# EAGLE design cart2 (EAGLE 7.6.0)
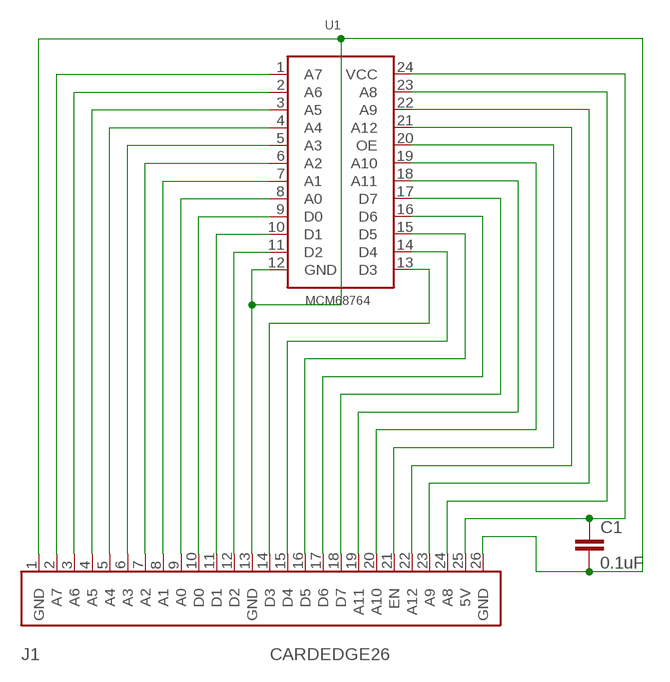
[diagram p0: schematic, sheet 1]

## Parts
C1  0.1uF  C-EU150-054X183  [C150-054X183]
J1  CARDEDGE26  [CARDEDGE26]
U1  MCM68764  [DIL24]

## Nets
GND: C1.2 J1.1(GND) J1.13(GND) J1.26(GND) U1.12(GND)
N$2: J1.2(A7) U1.1(A7)
N$3: J1.3(A6) U1.2(A6)
N$4: J1.4(A5) U1.3(A5)
N$5: J1.5(A4) U1.4(A4)
N$6: J1.6(A3) U1.5(A3)
N$7: J1.7(A2) U1.6(A2)
N$8: J1.8(A1) U1.7(A1)
N$9: J1.9(A0) U1.8(A0)
N$10: J1.10(D0) U1.9(D0)
N$11: J1.11(D1) U1.10(D1)
N$12: J1.12(D2) U1.11(D2)
N$13: J1.14(D3) U1.13(D3)
N$14: J1.15(D4) U1.14(D4)
N$15: J1.16(D5) U1.15(D5)
N$16: J1.17(D6) U1.16(D6)
N$17: J1.18(D7) U1.17(D7)
N$18: J1.19(A11) U1.18(A11)
N$19: J1.20(A10) U1.19(A10)
N$20: J1.21(EN) U1.20(OE)
N$21: J1.22(A12) U1.21(A12)
N$22: J1.23(A9) U1.22(A9)
N$23: J1.24(A8) U1.23(A8)
N$24: C1.1 J1.25(5V) U1.24(VCC)

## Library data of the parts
C1 = rcl:C-EU: CAPACITOR, European symbol
J1 = bally:CARDEDGE26: Bally Astrocade cartridge 26 pin card edge connector.
U1 = bally:MCM68764: Motorola MCM68764 EPROM (8K x 8)

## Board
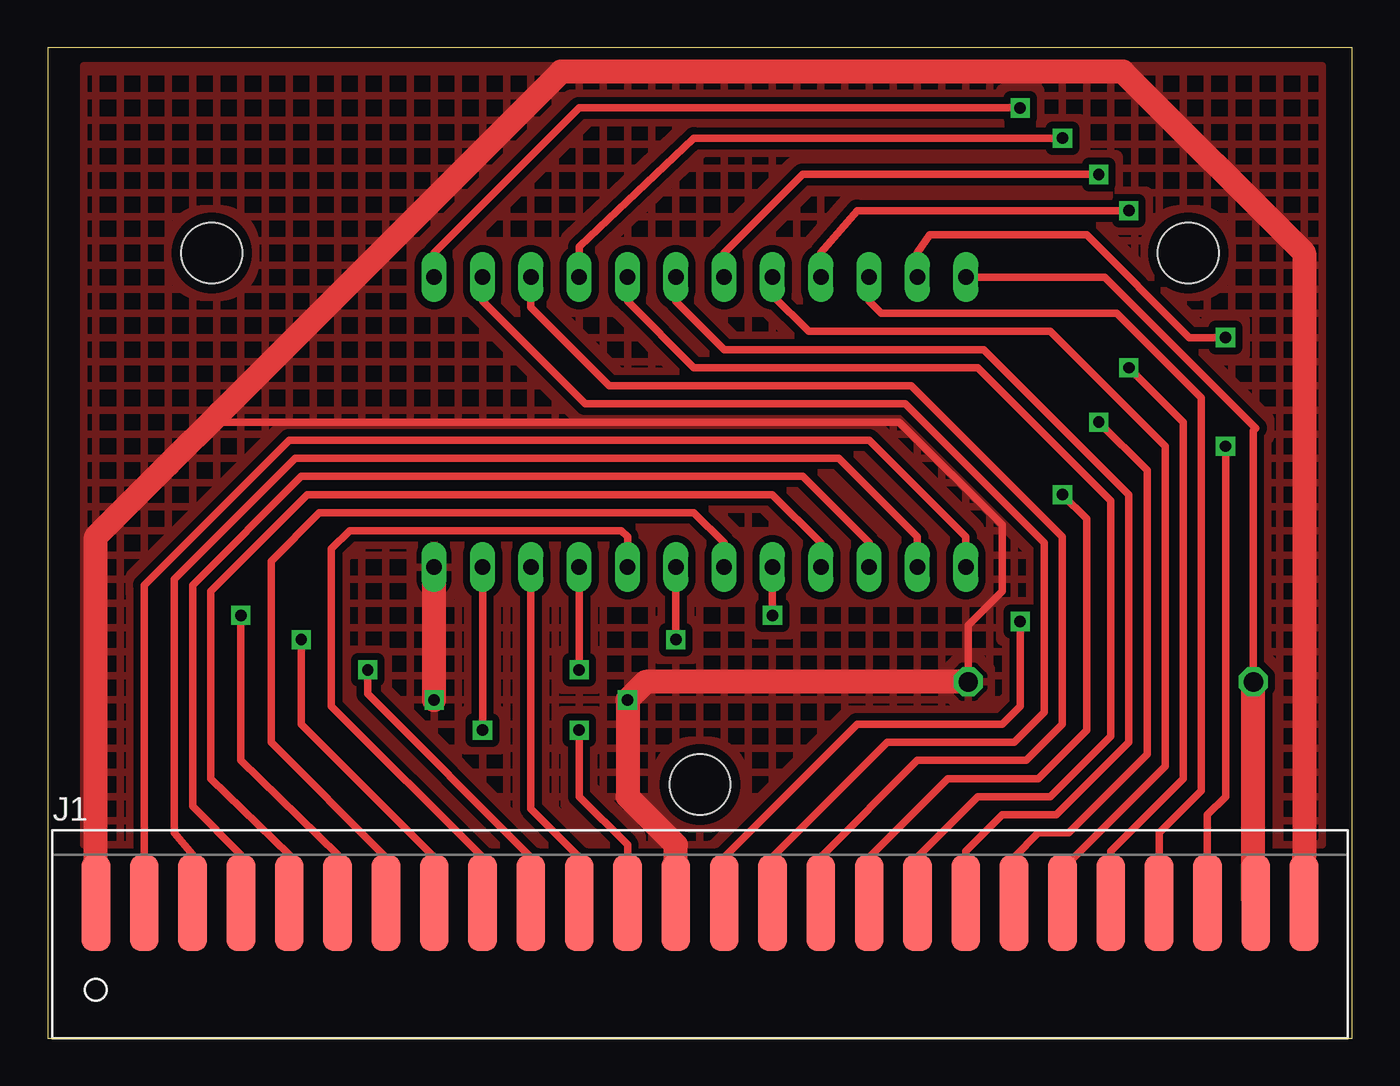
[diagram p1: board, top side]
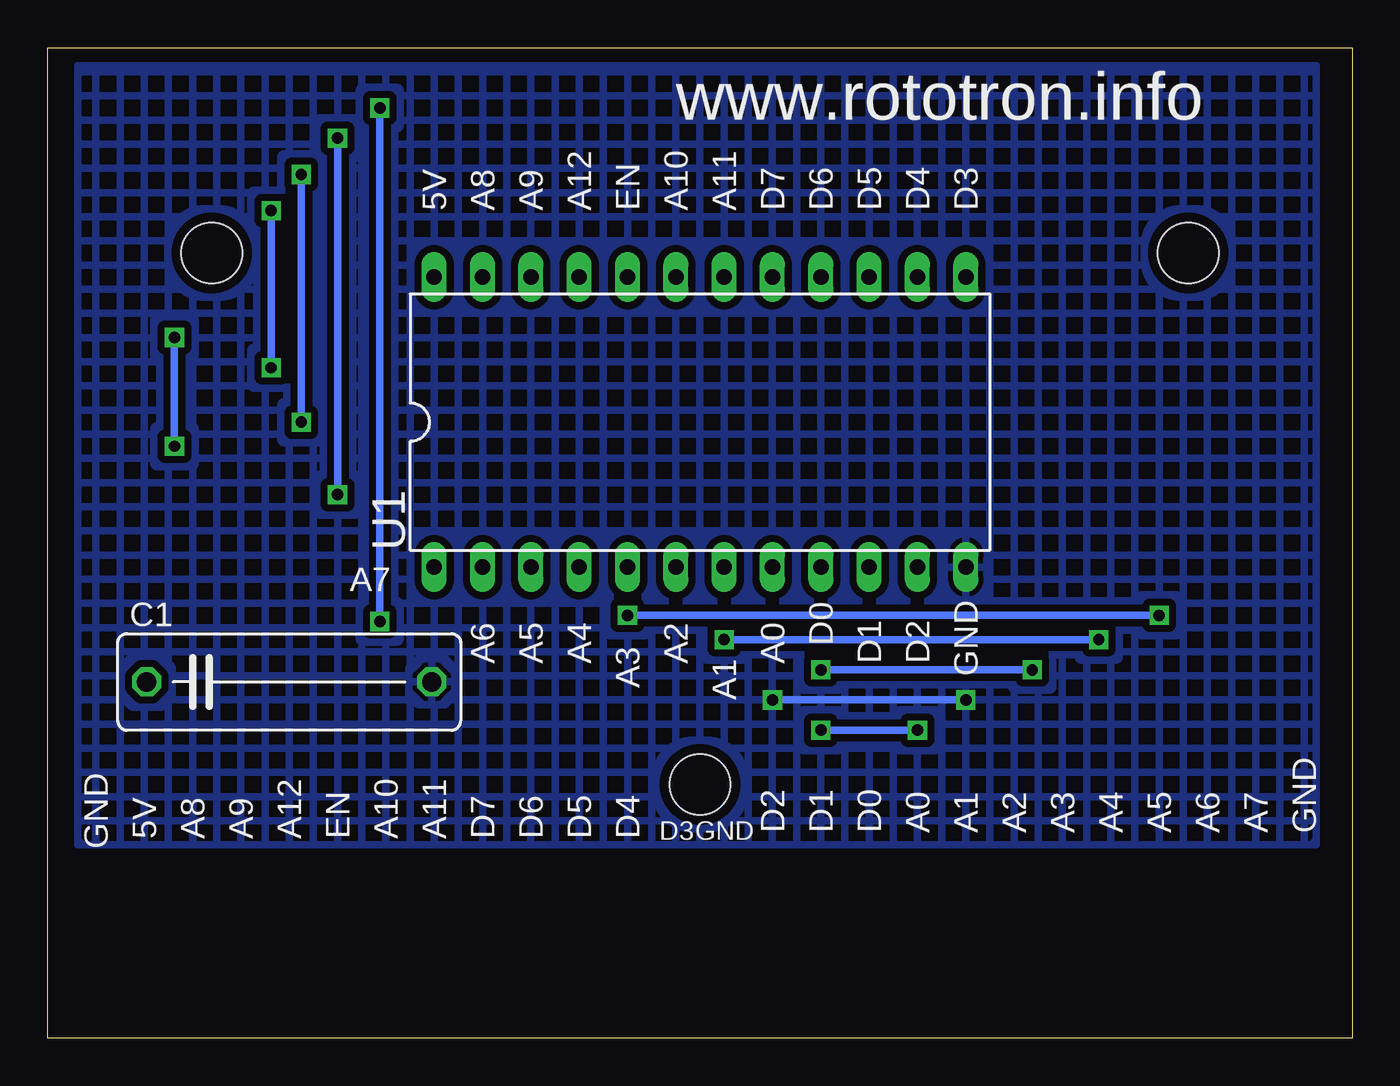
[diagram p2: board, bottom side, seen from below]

Size 68.58 x 52.06 mm. Coordinates in mm from the lower left corner, seen from the top.
Outline: 0,0 68.58,0 68.58,52.06 0,52.06 0,0
Copper layers (1*16): Top 0.035mm / dielectric 1.5mm / Bottom 0.035mm
Design rules "default *": minimum track width 10mil, minimum drill 24mil, track to track 15mil, track to pad 15mil, pad to pad 20mil, via to via 20mil, smd to smd 20mil, copper to edge 20mil, drill to drill 8mil, minimum pad ring 10mil, minimum via ring 8mil, stop-mask expansion 4mil, vias tented up to drill 0mil, thermal gap 10mil
Holes 3.2 mm at 34.29,13.34 8.64,41.27 59.94,41.27

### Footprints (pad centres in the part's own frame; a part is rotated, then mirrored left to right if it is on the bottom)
C150-054X183 = drill 1.016 octagon: 1 -7.493,0; 2 7.493,0
CARDEDGE26 = smd 1.524 x 5.08: 1 2.286,7.112; 2 4.826,7.112; 3 7.366,7.112; 4 9.906,7.112; 5 12.446,7.112; 6 14.986,7.112; 7 17.526,7.112; 8 20.066,7.112; 9 22.606,7.112; 10 25.146,7.112; 11 27.686,7.112; 12 30.226,7.112; 13 32.766,7.112; 14 35.306,7.112; 15 37.846,7.112; 16 40.386,7.112; 17 42.926,7.112; 18 45.466,7.112; 19 48.006,7.112; 20 50.546,7.112; 21 53.086,7.112; 22 55.626,7.112; 23 58.166,7.112; 24 60.706,7.112; 25 63.246,7.112; 26 65.786,7.112
DIL24 = drill 0.813 long: 1 1.27,-0.635; 2 3.81,-0.635; 3 6.35,-0.635; 4 8.89,-0.635; 5 11.43,-0.635; 6 13.97,-0.635; 7 16.51,-0.635; 8 19.05,-0.635; 9 21.59,-0.635; 10 24.13,-0.635; 11 26.67,-0.635; 12 29.21,-0.635; 13 29.21,14.605; 14 26.67,14.605; 15 24.13,14.605; 16 21.59,14.605; 17 19.05,14.605; 18 16.51,14.605; 19 13.97,14.605; 20 11.43,14.605; 21 8.89,14.605; 22 6.35,14.605; 23 3.81,14.605; 24 1.27,14.605

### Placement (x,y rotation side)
C1  55.88,18.73 0 bottom
J1  0.25,0 0 top
U1  49.53,25.4 0 bottom

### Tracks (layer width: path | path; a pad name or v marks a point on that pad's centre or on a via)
GND  (via drill 0.6)
  Top 0.406: 33.02,6.99 J1.13 | 66.04,9.53 J1.26 | 8.57,32.38 44.77,32.38 50.16,26.99 50.16,23.5 48.39,21.72 C1.2 | 8.57,32.38 8.61,32.35 | 8.57,32.38 8.26,32.07 9.05,32.86
  Top 1.27: J1.1 2.54,26.35 6.35,30.16 9.05,32.86 26.99,50.8 56.52,50.8 66.04,41.27 66.04,9.53 | v20.32,17.78 U1.12 | J1.13 33.02,10.16 30.48,12.7 v30.48,17.78 31.43,18.73 C1.2
  Bottom 0.406: v30.48,17.78 v20.32,17.78
  pour Top (hatched): 1.91,10.16 1.91,51.12 66.99,51.12 66.99,10.16
  pour Bottom (hatched): 1.91,10.16 1.91,51.12 66.99,51.12 66.99,10.16
N$2
  Top 0.406: U1.1 48.26,26.35 43.18,31.43 12.7,31.43 5.08,23.81 J1.2
N$3
  Top 0.406: U1.2 45.72,26.35 41.59,30.48 13.02,30.48 6.67,24.13 6.67,10.79 7.62,9.65 J1.3
N$4
  Top 0.406: U1.3 43.18,26.04 39.69,29.53 13.34,29.53 7.62,23.81 7.62,12.19 10.16,9.65 J1.4
N$5
  Top 0.406: U1.4 40.64,26.04 38.1,28.57 13.65,28.57 8.57,23.5 8.57,13.65 12.7,9.65 J1.5
N$6  (via drill 0.6)
  Top 0.406: U1.5 v38.1,22.23 | v10.16,22.23 10.16,14.61 15.24,9.65 J1.6
  Bottom 0.406: v38.1,22.23 v10.16,22.23
N$7
  Top 0.406: U1.6 35.56,26.04 33.97,27.62 14.29,27.62 11.75,25.08 11.75,15.56 17.78,9.53 J1.7
N$8  (via drill 0.6)
  Top 0.406: U1.7 v33.02,20.95 | v13.34,20.95 13.34,16.51 20.32,9.53 J1.8
  Bottom 0.406: v33.02,20.95 v13.34,20.95
N$9
  Top 0.406: U1.8 30.48,26.35 30.16,26.67 15.88,26.67 14.92,25.72 14.92,17.46 22.86,9.53 J1.9
N$10  (via drill 0.6)
  Top 0.406: U1.9 v27.94,19.37 | v16.83,19.37 16.83,18.1 25.4,9.53 J1.10
  Bottom 0.406: v27.94,19.37 v16.83,19.37
N$11
  Top 0.406: U1.10 25.4,12.06 27.94,9.53 J1.11
N$12  (via drill 0.6)
  Top 0.406: J1.12 30.48,10.16 27.94,12.7 v27.94,16.19 | v22.86,16.19 U1.11
  Bottom 0.406: v27.94,16.19 v22.86,16.19
N$13  (via drill 0.6)
  Top 0.406: U1.13 20.32,41.27 27.94,48.9 v51.12,48.9 | v51.12,21.91 51.12,17.46 50.16,16.51 42.55,16.51 35.56,9.53 J1.14
  Bottom 0.406: v51.12,48.9 v51.12,21.91
N$14
  Top 0.406: U1.14 22.86,38.73 28.26,33.34 45.09,33.34 52.39,26.04 52.39,17.14 50.8,15.56 44.13,15.56 38.1,9.53 J1.15
N$15
  Top 0.406: U1.15 25.4,38.42 29.53,34.29 45.4,34.29 53.34,26.35 53.34,16.51 51.44,14.61 45.72,14.61 40.64,9.53 J1.16
N$16  (via drill 0.6)
  Top 0.406: U1.16 27.94,41.59 33.97,47.31 v53.34,47.31 | v53.34,28.57 54.61,27.3 54.61,16.19 52.07,13.65 47.31,13.65 43.18,9.53 J1.17
  Bottom 0.406: v53.34,47.31 v53.34,28.57
N$17
  Top 0.406: U1.17 30.48,38.73 33.97,35.24 48.9,35.24 55.88,28.26 55.88,15.88 52.7,12.7 48.9,12.7 45.72,9.53 J1.18
N$18
  Top 0.406: U1.18 33.02,38.73 35.56,36.2 49.21,36.2 56.83,28.57 56.83,15.56 53.02,11.75 50.16,11.75 48.26,9.84 J1.19
N$19  (via drill 0.6)
  Top 0.406: U1.19 35.56,41.27 39.69,45.4 v55.24,45.4 | v55.24,32.38 57.78,29.84 57.78,14.92 53.66,10.79 52.07,10.79 50.8,9.53 J1.20
  Bottom 0.406: v55.24,45.4 v55.24,32.38
N$20
  Top 0.406: U1.20 38.1,39.05 40.01,37.15 52.7,37.15 58.74,31.11 58.74,14.29 53.34,8.89 J1.21
N$21  (via drill 0.6)
  Top 0.406: U1.21 40.64,41.27 42.55,43.5 v56.83,43.5 | v56.83,35.24 59.69,32.38 59.69,13.65 55.88,9.84 J1.22
  Bottom 0.406: v56.83,43.5 v56.83,35.24
N$22
  Top 0.406: U1.22 43.18,38.73 43.81,38.1 56.2,38.1 60.64,33.66 60.64,13.02 58.42,10.79 J1.23
N$23  (via drill 0.6)
  Top 0.406: U1.23 45.72,41.27 46.35,42.23 54.61,42.23 60.01,36.83 v61.91,36.83 | J1.24 60.96,11.75 61.91,12.7 v61.91,31.11
  Bottom 0.406: v61.91,36.83 v61.91,31.11
N$24
  Top 0.406: U1.24 55.56,40.01 63.5,32.07 63.37,31.94 C1.1
  Top 1.27: J1.25 63.37,7.24 C1.1

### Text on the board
bNames: www.rototron.info | D3 | D4 | D5 | D6 | D7 | A11 | A10 | EN | A12 | A9 | A8 | 5V | A7 | D0 | D2 | D1 | A0 | A2 | A4 | A5 | A6 | GND | A1 | A3 | GND | GND | A7 | A6 | A5 | A4 | A3 | A2 | A1 | A0 | D0 | D1 | D2 | GND | D3 | D4 | D5 | D6 | D7 | A11 | A10 | EN | A12 | A9 | A8 | 5V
